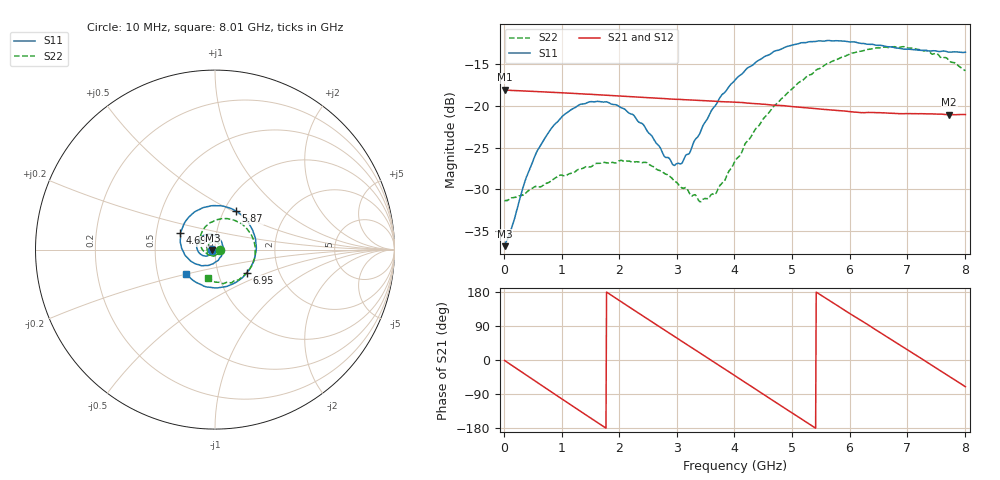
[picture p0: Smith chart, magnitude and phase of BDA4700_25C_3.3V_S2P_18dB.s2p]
!Agilent Technologies,E5071B,MY42404982,A.09.10
!Date: Mon Oct 20 18:10:36 2025
!Data & Calibration Information:
!Freq	S11:SOLT2(ON)	S21:SOLT2(ON)	S12:SOLT2(ON)	S22:SOLT2(ON)
# Hz S RI R 50
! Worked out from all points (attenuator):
!   801 points, 10 MHz to 8.01 GHz, reference 50 ohm
!   highest |S21| = -18.08 dB at 10 MHz (marker M1); lowest = -21.1 dB at 7.73 GHz (marker M2)
!   lowest |S11| = -36.8 dB at 10 MHz (marker M3), VSWR 1.03, Z = 48.6 - j0.129 ohm
!   |S11| at or under -10 dB: start of sweep to end of sweep
!   |S22| runs from -31.5 to -12.9 dB; largest |S21 - S12| = 0.0014
!   S11 on the Smith chart (normalised r, x): 10 MHz: 0.97, -0.00; 4.69 GHz: 0.67, +0.13; 5.87 GHz: 1.14, +0.52; 6.95 GHz: 1.37, -0.37; 8.01 GHz: 0.70, -0.20
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1e7  -0.0143 -0.00132  0.1247 -0.00267  0.1246 -0.00279  0.027 -0.00084
3.8e8  -0.0255 -0.0263  0.0949 -0.0778  0.0948 -0.0778  0.0218 -0.0207
5.9e8  -0.0418 -0.0354  0.0595 -0.1062  0.0595 -0.1062  0.0134 -0.0299
1e9  -0.082 -0.0243  -0.0254 -0.117  -0.0254 -0.1171  -0.0162 -0.0349
1.35e9  -0.1019 0.0118  -0.0872 -0.0796  -0.0872 -0.0797  -0.0385 -0.0168
2.07e9  -0.0449 0.0853  -0.0991 0.0567  -0.0991 0.0568  -0.0286 0.0369
2.68e9  0.0357 0.0457  0.000667 0.111  0.000516 0.111  0.018 0.0369
2.94e9  0.044 0.00308  0.048 0.0987  0.048 0.0984  0.0293 0.0208
3.08e9  0.0397 -0.0213  0.0702 0.0836  0.0693 0.084  0.0311 0.00882
3.4e9  0.0039 -0.0682  0.1021 0.0344  0.1022 0.0346  0.0214 -0.0159
3.54e9  -0.0208 -0.0823  0.1068 0.00911  0.1068 0.00894  0.0122 -0.0251
3.69e9  -0.0524 -0.0884  0.1048 -0.0182  0.1049 -0.0186  -0.00185 -0.0303
4.01e9  -0.1236 -0.0711  0.0786 -0.0699  0.0787 -0.0697  -0.0367 -0.0285
4.69e9  -0.1922 0.0904  -0.033 -0.0954  -0.0326 -0.0956  -0.0849 0.0526
5.35e9  -0.0561 0.2363  -0.0962 -0.01  -0.0961 -0.0106  -0.0138 0.1549
5.87e9  0.1183 0.2137  -0.0667 0.0654  -0.0665 0.0652  0.109 0.1631
6.27e9  0.2099 0.1079  -0.0125 0.0902  -0.0112 0.0902  0.1925 0.0971
6.68e9  0.2225 -0.0405  0.0479 0.0766  0.0482 0.0766  0.2239 -0.0102
6.95e9  0.1774 -0.128  0.0758 0.0481  0.0761 0.0475  0.2094 -0.0852
7.33e9  0.062 -0.2058  0.0892 -0.00698  0.0893 -0.00704  0.1359 -0.166
7.73e9  -0.0831 -0.1928  0.0643 -0.0607  0.0644 -0.0609  0.0293 -0.184
8.01e9  -0.1617 -0.1333  0.0295 -0.0836  0.0298 -0.0836  -0.0414 -0.157
